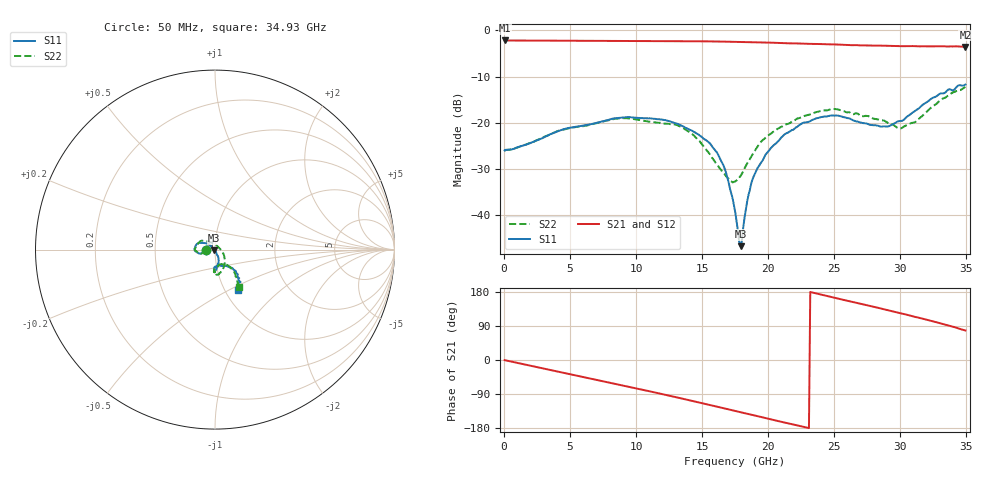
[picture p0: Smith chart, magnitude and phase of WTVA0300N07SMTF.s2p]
! 50 ohm 2-Port S-parameters measured by Modelithics Inc support@modelithics.com  Tampa, FL USA 813-866-6335 (February 2024)
! Smiths Interconnect,  3dB P/N: WTVA0300N07SMTF, Temperature: 75 C
! Board: 10 mil Rogers 4350B, Mounting Pad Dimensions: Length: 15 mils, Width: 25 mils, Gap: 40 mils.
# Hz S RI R 50
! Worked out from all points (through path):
!   352 points, 50 MHz to 34.93 GHz, reference 50 ohm
!   highest |S21| = -2.17 dB at 100 MHz (marker M1); lowest = -3.6 dB at 34.93 GHz (marker M2)
!   group delay of S21, straight-line fit = 22.2 ps
!   lowest |S11| = -46.7 dB at 17.91 GHz (marker M3), VSWR 1.01, Z = 49.6 - j0.281 ohm
!   |S11| at or under -10 dB: start of sweep to end of sweep
!   |S22| runs from -32.9 to -12.2 dB; largest |S21 - S12| = 0.0092
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5e7  -0.0502 0.000366  0.779 -0.00457  0.778 -0.00461  -0.0494 -0.000815
1e8  -0.0508 -0.000614  0.779 -0.0104  0.7781 -0.0105  -0.0505 -0.00111
2.787e9  -0.0655 -0.0149  0.7258 -0.2749  0.7247 -0.2749  -0.0657 -0.0161
5.8715e9  -0.0903 -0.0206  0.5581 -0.5339  0.5573 -0.5335  -0.0892 -0.0192
8.956e9  -0.1141 -0.00264  0.3018 -0.7065  0.3005 -0.7058  -0.1122 0.000461
1.1742e10  -0.1066 0.0239  0.0245 -0.7658  0.0227 -0.7648  -0.0945 0.0334
1.36325e10  -0.0821 0.0377  -0.1728 -0.7455  -0.174 -0.7443  -0.0707 0.0496
1.56225e10  -0.0477 0.035  -0.3699 -0.6647  -0.3712 -0.6628  -0.0207 0.0398
1.6717e10  -0.0229 0.0218  -0.4656 -0.5965  -0.4664 -0.5948  0.00486 0.0272
1.7513e10  -0.00981 0.00408  -0.5283 -0.5379  -0.5284 -0.5364  0.0185 0.0139
1.78115e10  -0.00493 -0.00114  -0.5505 -0.5122  -0.5497 -0.5115  0.024 0.00892
1.7911e10  -0.00363 -0.00283  -0.5572 -0.5036  -0.5564 -0.503  0.0256 0.00682
1.8508e10  0.006 -0.0154  -0.5939 -0.4535  -0.5942 -0.4521  0.0372 -0.0085
1.92045e10  0.0117 -0.0304  -0.6329 -0.3902  -0.6322 -0.3899  0.0486 -0.027
2.11945e10  0.0201 -0.0712  -0.7024 -0.1924  -0.7016 -0.1915  0.0546 -0.0762
2.33835e10  0.00844 -0.1077  -0.7151 0.0274  -0.7143 0.0276  0.0332 -0.1224
2.5274e10  -0.00388 -0.1195  -0.669 0.2171  -0.6681 0.217  0.00709 -0.1394
2.91545e10  0.025 -0.0884  -0.4439 0.5176  -0.4379 0.5213  0.00885 -0.0974
3.005e10  0.0511 -0.0912  -0.3664 0.5677  -0.3624 0.5693  0.0307 -0.0813
3.11445e10  0.0896 -0.1016  -0.2683 0.6178  -0.2666 0.6175  0.0595 -0.083
3.3035e10  0.1341 -0.1583  -0.0794 0.6691  -0.0732 0.6689  0.1128 -0.1362
3.49255e10  0.1297 -0.2251  0.1392 0.6477  0.1399 0.6463  0.1332 -0.2056
